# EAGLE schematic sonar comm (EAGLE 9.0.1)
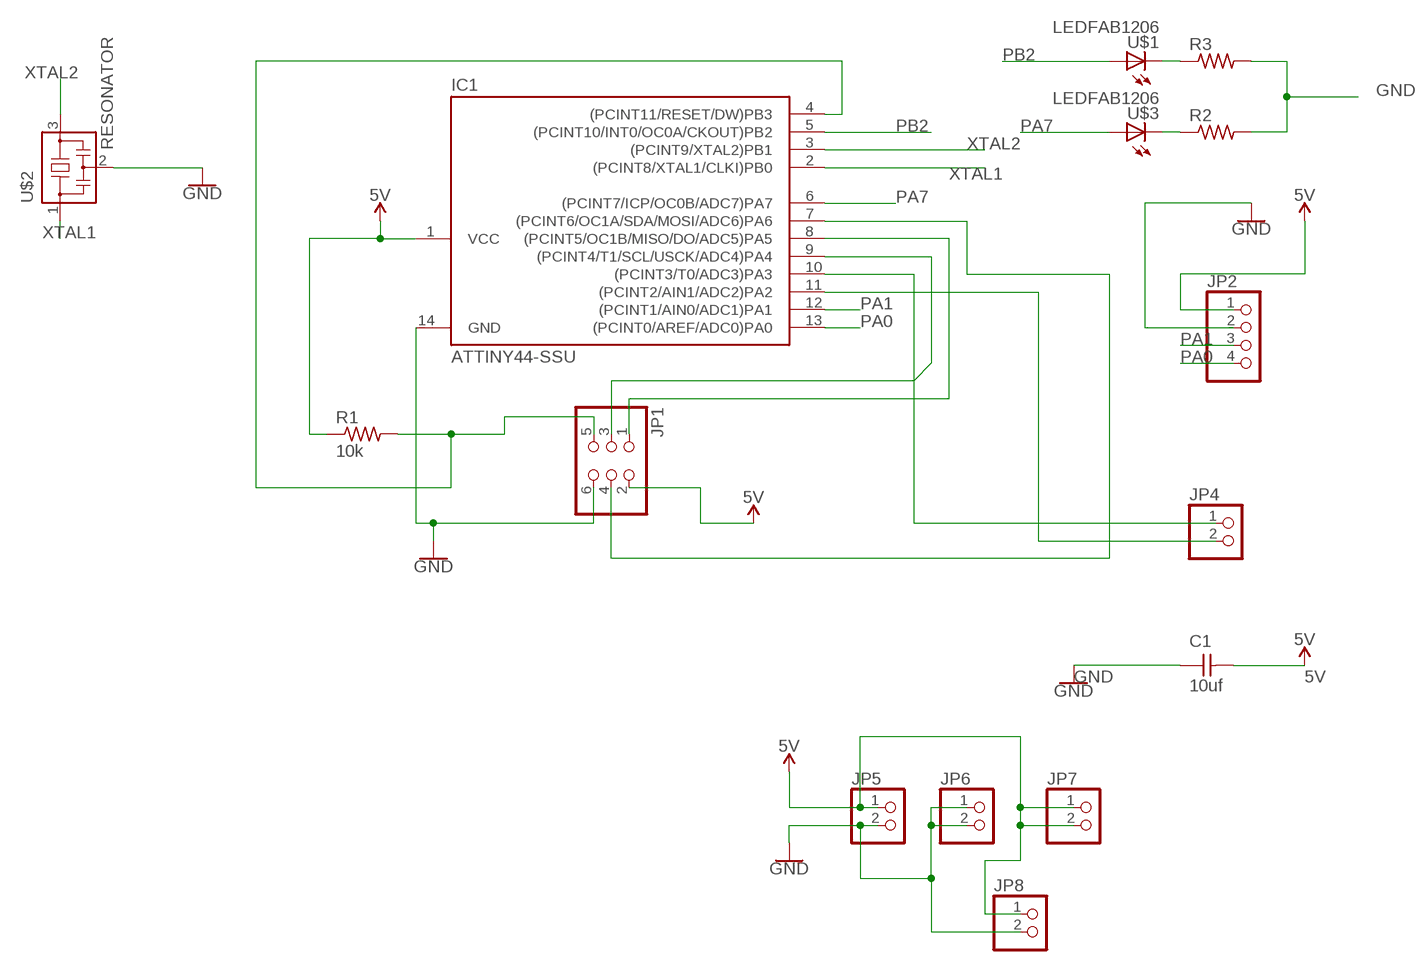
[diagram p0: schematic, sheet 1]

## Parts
C1  10uf  CAP-UNPOLARIZEDFAB  [C1206FAB]
IC1  ATTINY44-SSU  [SOIC14]
JP1  PINHD-2X3-SMD  [2X03SMD]
JP2  PINHD-1X4  [1X04]
JP4  PINHD-1X2  [1X02]
JP5  PINHD-1X2  [1X02]
JP6  PINHD-1X2  [1X02]
JP7  PINHD-1X2  [1X02]
JP8  PINHD-1X2  [1X02]
R1  10k  RES-US1206FAB  [R1206FAB]
R2  RES-US1206FAB  [R1206FAB]
R3  RES-US1206FAB  [R1206FAB]
U$1  LEDFAB1206  [LED1206FAB]
U$2  RESONATOR  [EFOBM]
U$3  LEDFAB1206  [LED1206FAB]

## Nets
5V: C1.2 IC1.1(VCC) JP1.2 JP2.1 JP5.1 JP7.1 JP7.2 JP8.1 R1.1
GND: C1.1 IC1.14(GND) JP1.6 JP2.2 JP5.2 JP6.1 JP6.2 JP8.2 R2.2 R3.2 U$2.2
N$3: IC1.11((PCINT2/AIN1/ADC2)PA2) JP4.2
N$4: IC1.7((PCINT6/OC1A/SDA/MOSI/ADC6)PA6) JP1.4
N$5: IC1.4((PCINT11/RESET/DW)PB3) JP1.5 R1.2
N$6: IC1.9((PCINT4/T1/SCL/USCK/ADC4)PA4) JP1.3
N$7: IC1.8((PCINT5/OC1B/MISO/DO/ADC5)PA5) JP1.1
N$10: IC1.10((PCINT3/T0/ADC3)PA3) JP4.1
N$13: R3.1 U$1.2(C)
N$14: R2.1 U$3.2(C)
PA0: IC1.13((PCINT0/AREF/ADC0)PA0) JP2.4
PA1: IC1.12((PCINT1/AIN0/ADC1)PA1) JP2.3
PA7: IC1.6((PCINT7/ICP/OC0B/ADC7)PA7) U$3.1(A)
PB2: IC1.5((PCINT10/INT0/OC0A/CKOUT)PB2) U$1.1(A)
XTAL1: IC1.2((PCINT8/XTAL1/CLKI)PB0) U$2.1
XTAL2: IC1.3((PCINT9/XTAL2)PB1) U$2.3

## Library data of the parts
C1 = fab:CAP-UNPOLARIZED
IC1 = fab:ATTINY44
JP1 = fab:PINHD-2X3-SMD: PIN HEADER
JP2 = pinhead:PINHD-1X4: PIN HEADER
JP4-JP8 = pinhead:PINHD-1X2: PIN HEADER
R1-R3 = fab:RES-US: Resistor (US Symbol)
U$1 U$3 = fab:LED: LED
U$2 = fab:RESONATOR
